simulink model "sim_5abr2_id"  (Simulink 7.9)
settings: Solver=ode45  StartTime=0.0  StopTime=2  RelTol=1e-3  AbsTol=1e-3
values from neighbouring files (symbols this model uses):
  m = 1    [mechanical_system.m]
  s = Lv/norm(Lv)    [pkm1.m]
undefined symbols (not defined in the file or in its folder): deg, kg, mN, N, rad
libraries: mblibv1 x16

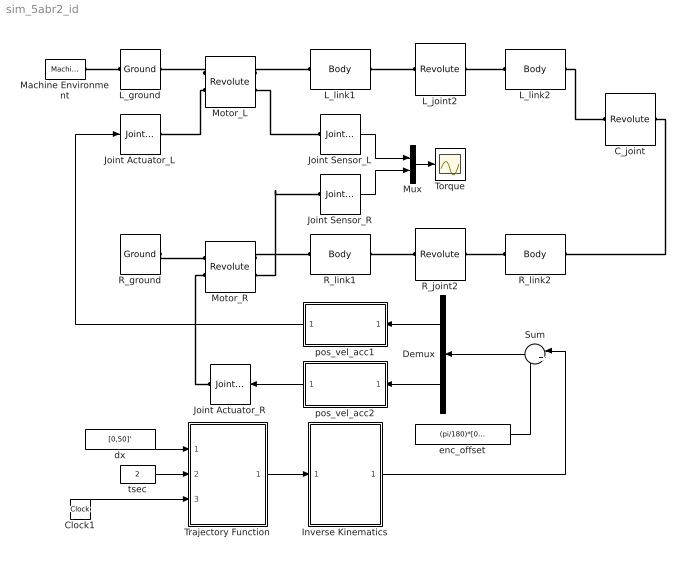
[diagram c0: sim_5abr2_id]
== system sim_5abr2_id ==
  C_joint : mblibv1/Joints/Revolute  LConnTagsString=__newl0  RConnTagsString=__newr0  UpdateFromCAD=off  NumSAPorts=0  CutJoint=off  MarkAsCut=off  Primitives=prismatic  PrimitiveProps=R1$World$[0 0 1]$revolute  DialogClass=JointBlock  R1Axis=[0 0 1]
  Clock1 : Clock
  Demux : Demux  Outputs=2
  Inverse Kinematics : MATLAB Function  TreatAsAtomicUnit=on
  Joint Actuator_L : mblibv1/Sensors &  Actuators/Joint Actuator  UpdateFromCAD=off  PhysicalDomain=Mechanical  PortType=blob  ActuationStyle=Motion  AngleUnits=rad  ArcVelocityUnits=rad/s  ArcAccelerationUnits=rad/s^2  CoordPositionUnits=m  VelocityUnits=m/s  AccelerationUnits=m/s^2  ForceUnits=N  TorqueUnits=N*m  ActiveIO=on  Width=3  DialogClass=MechanicalActuatorBlock  Primitive=R1  ReferenceFrame=Absolute (World)
  Joint Actuator_R : mblibv1/Sensors &  Actuators/Joint Actuator  UpdateFromCAD=off  PhysicalDomain=Mechanical  PortType=blob  ActuationStyle=Motion  AngleUnits=rad  ArcVelocityUnits=rad/s  ArcAccelerationUnits=rad/s^2  CoordPositionUnits=m  VelocityUnits=m/s  AccelerationUnits=m/s^2  ForceUnits=N  TorqueUnits=N*m  ActiveIO=on  Width=3  DialogClass=MechanicalActuatorBlock  Primitive=R1  ReferenceFrame=Absolute (World)
  Joint Sensor_L : mblibv1/Sensors &  Actuators/Joint Sensor  UpdateFromCAD=off  PhysicalDomain=Mechanical  PortType=blob  Muxed=on  Pose=off  Angle=off  AngleUnits=deg  ArcVelocity=off  ArcVelocityUnits=deg/s  ArcAcceleration=off  ArcAccelerationUnits=deg/s^2  CoordPosition=on  CoordPositionUnits=m  Velocity=off  VelocityUnits=m/s  Acceleration=off  AccelerationUnits=m/s^2  Quaternion=on  QuaternionDT=off  QuaternionDDT=off  QuaternionUnits=off  OutputVector=[1]  ActiveIO=on  Width=1  DialogClass=MechanicalSensorBlock  Primitive=R1  Force=off  ForceUnits=N  Torque=on  TorqueUnits=mN*m  ReferenceFrame=Absolute (World)  ReactionSensedSide=Base  ReactionReferenceFrame=Absolute (World)  ReactionForce=off  ReactionForceUnits=N  ReactionMoment=off  ReactionMomentUnits=N*m
  Joint Sensor_R : mblibv1/Sensors &  Actuators/Joint Sensor  UpdateFromCAD=off  PhysicalDomain=Mechanical  PortType=blob  Muxed=on  Pose=off  Angle=off  AngleUnits=deg  ArcVelocity=off  ArcVelocityUnits=deg/s  ArcAcceleration=off  ArcAccelerationUnits=deg/s^2  CoordPosition=on  CoordPositionUnits=m  Velocity=off  VelocityUnits=m/s  Acceleration=off  AccelerationUnits=m/s^2  Quaternion=on  QuaternionDT=off  QuaternionDDT=off  QuaternionUnits=off  OutputVector=[1]  ActiveIO=on  Width=1  DialogClass=MechanicalSensorBlock  Primitive=R1  Force=off  ForceUnits=N  Torque=on  TorqueUnits=mN*m  ReferenceFrame=Absolute (World)  ReactionSensedSide=Base  ReactionReferenceFrame=Absolute (World)  ReactionForce=off  ReactionForceUnits=N  ReactionMoment=off  ReactionMomentUnits=N*m
  L_ground : mblibv1/Bodies/Ground  UpdateFromCAD=off  LeftPortType=env  RightPortType=workingframe  PhysicalDomain=Mechanical  DialogClass=GroundBlock  CoordPosition=[0 0 0]  CoordPositionUnits=cm  StateVectorMgrId=-1  MachineId=[0 0]  ShowEnvPort=on
  L_joint2 : mblibv1/Joints/Revolute  LConnTagsString=__newl0  RConnTagsString=__newr0  UpdateFromCAD=off  NumSAPorts=0  CutJoint=off  MarkAsCut=off  Primitives=prismatic  PrimitiveProps=R1$World$[0 0 1]$revolute  DialogClass=JointBlock  R1Axis=[0 0 1]
  L_link1 : mblibv1/Bodies/Body  LConnTagsString=CS1  RConnTagsString=CS2  UpdateFromCAD=off  DialogClass=MechanicalBodyBlock  Mass=0.053  MassUnits=kg  InertiaUnits=kg*m^2  Inertia=[0.000110621 0 0; 0 0.000110621 0; 0 0 0]  Shape=Cylinder  ShapeDims=[1 1]  ShapeUnits=m  ShapeUse=false  Density=1  DensityUnits=kg/m^3  DensityUse=false  GraphicsMode=MACHINE_DEFAULT  BodyColorSelMode=MACHINE_DEFAULT  BodyColor=[1 0 0]  AttachedToCS=CG  CG=Left$CG$[0.05311 0 0]$CS1$CS1$m$[0 0 0]$Euler X-Y-Z$deg$WORLD$false$none  WorkingFrames=Left$CS1$[0 0 0]$World$World$m$[0 0 0]$Euler X-Y-Z$deg$WORLD$true$none#Right$CS2$[0.1 0 0]$World$World$m$[0 0 0]$Euler X-Y-Z$deg$WORLD$true$none  CGPos=[0.05311 0 0]  CGRot=[0 0 0]  CS0Pos=[]  CS0Rot=[]  CS1Pos=[0 0 0]  CS1Rot=[0 0 0]  CS2Pos=[0.1 0 0]  CS2Rot=[0 0 0]  CS3Pos=[]  CS3Rot=[]  CS4Pos=[]  CS4Rot=[]  CS5Pos=[]  CS5Rot=[]  CS6Pos=[]  CS6Rot=[]  CS7Pos=[]  CS7Rot=[]  CS8Pos=[]  CS8Rot=[]  CS9Pos=[]  CS9Rot=[]  CS10Pos=[]  CS10Rot=[]  CS11Pos=[]  CS11Rot=[]  CS12Pos=[]  CS12Rot=[]  CS13Pos=[]  CS13Rot=[]  CS14Pos=[]  CS14Rot=[]  CS15Pos=[]  CS15Rot=[]  CS16Pos=[]  CS16Rot=[]  CS17Pos=[]  CS17Rot=[]  CS18Pos=[]  CS18Rot=[]  CS19Pos=[]  CS19Rot=[]  CS20Pos=[]  CS20Rot=[]
  L_link2 : mblibv1/Bodies/Body  LConnTagsString=CS1  RConnTagsString=CS2  UpdateFromCAD=off  DialogClass=MechanicalBodyBlock  Mass=0.054  MassUnits=kg  InertiaUnits=kg*m^2  Inertia=[0.000120188 0 0; 0 0.000120188 0; 0 0 0]  Shape=Cylinder  ShapeDims=[1 1]  ShapeUnits=m  ShapeUse=false  Density=1  DensityUnits=kg/m^3  DensityUse=false  GraphicsMode=MACHINE_DEFAULT  BodyColorSelMode=MACHINE_DEFAULT  BodyColor=[1 0 0]  AttachedToCS=CG  CG=Left$CG$[0 0.05992 0]$CS1$CS1$m$[0 0 0]$Euler X-Y-Z$deg$WORLD$false$none  WorkingFrames=Left$CS1$[0.1 0 0]$World$World$m$[0 0 0]$Euler X-Y-Z$deg$WORLD$true$none#Right$CS2$[0.1 0.1 0]$World$World$m$[0 0 0]$Euler X-Y-Z$deg$WORLD$true$none#Left$CS3$[0.1 0.128 0]$World$World$m$[0 0 0]$Euler X-Y-Z$deg$WORLD$false$none  CGPos=[0 0.05992 0]  CGRot=[0 0 0]  CS0Pos=[]  CS0Rot=[]  CS1Pos=[0.1 0 0]  CS1Rot=[0 0 0]  CS2Pos=[0.1 0.1 0]  CS2Rot=[0 0 0]  CS3Pos=[0.1 0.128 0]  CS3Rot=[0 0 0]  CS4Pos=[]  CS4Rot=[]  CS5Pos=[]  CS5Rot=[]  CS6Pos=[]  CS6Rot=[]  CS7Pos=[]  CS7Rot=[]  CS8Pos=[]  CS8Rot=[]  CS9Pos=[]  CS9Rot=[]  CS10Pos=[]  CS10Rot=[]  CS11Pos=[]  CS11Rot=[]  CS12Pos=[]  CS12Rot=[]  CS13Pos=[]  CS13Rot=[]  CS14Pos=[]  CS14Rot=[]  CS15Pos=[]  CS15Rot=[]  CS16Pos=[]  CS16Rot=[]  CS17Pos=[]  CS17Rot=[]  CS18Pos=[]  CS18Rot=[]  CS19Pos=[]  CS19Rot=[]  CS20Pos=[]  CS20Rot=[]
  Machine Environment : mblibv1/Bodies/Machine Environment  PortType=env  PhysicalDomain=Mechanical  DialogTemplateClass=MECH.MachineEnvironment  SyncWhenCopied=off  Gravity=[0 -9.81 0]  GravityUnits=m/s^2  GravityAsSignal=off  Dimensionality=Auto-detect  AnalysisType=Forward dynamics  LinearAssemblyTolerance=1e-3  LinearAssemblyToleranceUnits=m  AngularAssemblyTolerance=1e-3  AngularAssemblyToleranceUnits=rad  ConstraintSolverType=Stabilizing  ConstraintRelTolerance=1e-4  ConstraintAbsTolerance=1e-4  UseRobustSingularityHandling=off  RedundancyAnalysisToleranceType=Automatically select tolerance  RedundancyAnalysisTolerance=1e-14  StatePerturbationType=Fixed  PerturbationSize=1e-5  VisualizeMachine=on  BodyVisualizationType=Use model default body geometries  BodyColorSelMode=Use model default  DefaultBodyColor=[1 0 0]
  Motor_L : mblibv1/Joints/Revolute  LConnTagsString=__newl0|SA1  RConnTagsString=__newr0|SA1  UpdateFromCAD=off  NumSAPorts=2  CutJoint=off  MarkAsCut=off  Primitives=prismatic  PrimitiveProps=R1$World$[0 0 1]$revolute  DialogClass=JointBlock  R1Axis=[0 0 1]
  Motor_R : mblibv1/Joints/Revolute  LConnTagsString=__newl0|SA1  RConnTagsString=__newr0|SA1  UpdateFromCAD=off  NumSAPorts=2  CutJoint=off  MarkAsCut=off  Primitives=prismatic  PrimitiveProps=R1$World$[0 0 1]$revolute  DialogClass=JointBlock  R1Axis=[0 0 1]
  Mux : Mux  Inputs=2
  R_ground : mblibv1/Bodies/Ground  UpdateFromCAD=off  LeftPortType=env  RightPortType=workingframe  PhysicalDomain=Mechanical  DialogClass=GroundBlock  CoordPosition=[0.2 0 0]  CoordPositionUnits=m  StateVectorMgrId=-1  MachineId=[0 0]  ShowEnvPort=off
  R_joint2 : mblibv1/Joints/Revolute  LConnTagsString=__newl0  RConnTagsString=__newr0  UpdateFromCAD=off  NumSAPorts=0  CutJoint=off  MarkAsCut=off  Primitives=prismatic  PrimitiveProps=R1$World$[0 0 1]$revolute  DialogClass=JointBlock  R1Axis=[0 0 1]
  R_link1 : mblibv1/Bodies/Body  LConnTagsString=CS1  RConnTagsString=CS2  UpdateFromCAD=off  DialogClass=MechanicalBodyBlock  Mass=0.061  MassUnits=kg  InertiaUnits=kg*m^2  Inertia=[0.000134303 0 0; 0 0.000134303 0; 0 0 0]  Shape=Cylinder  ShapeDims=[1 1]  ShapeUnits=m  ShapeUse=false  Density=1  DensityUnits=kg/m^3  DensityUse=false  GraphicsMode=MACHINE_DEFAULT  BodyColorSelMode=MACHINE_DEFAULT  BodyColor=[1 0 0]  AttachedToCS=CG  CG=Left$CG$[0 0.04569 0]$CS1$CS1$m$[0 0 0]$Euler X-Y-Z$deg$WORLD$false$none  WorkingFrames=Left$CS1$[0.2 0 0]$World$World$m$[0 0 0]$Euler X-Y-Z$deg$WORLD$true$none#Right$CS2$[0.2 0.1 0]$World$World$m$[0 0 0]$Euler X-Y-Z$deg$WORLD$true$none  CGPos=[0 0.04569 0]  CGRot=[0 0 0]  CS0Pos=[]  CS0Rot=[]  CS1Pos=[0.2 0 0]  CS1Rot=[0 0 0]  CS2Pos=[0.2 0.1 0]  CS2Rot=[0 0 0]  CS3Pos=[]  CS3Rot=[]  CS4Pos=[]  CS4Rot=[]  CS5Pos=[]  CS5Rot=[]  CS6Pos=[]  CS6Rot=[]  CS7Pos=[]  CS7Rot=[]  CS8Pos=[]  CS8Rot=[]  CS9Pos=[]  CS9Rot=[]  CS10Pos=[]  CS10Rot=[]  CS11Pos=[]  CS11Rot=[]  CS12Pos=[]  CS12Rot=[]  CS13Pos=[]  CS13Rot=[]  CS14Pos=[]  CS14Rot=[]  CS15Pos=[]  CS15Rot=[]  CS16Pos=[]  CS16Rot=[]  CS17Pos=[]  CS17Rot=[]  CS18Pos=[]  CS18Rot=[]  CS19Pos=[]  CS19Rot=[]  CS20Pos=[]  CS20Rot=[]
  R_link2 : mblibv1/Bodies/Body  LConnTagsString=CS1  RConnTagsString=CS2  UpdateFromCAD=off  DialogClass=MechanicalBodyBlock  Mass=0.045  MassUnits=kg  InertiaUnits=kg*m^2  Inertia=[0.000090992 0 0; 0 0.000090992 0; 0 0 0]  Shape=Cylinder  ShapeDims=[1 1]  ShapeUnits=m  ShapeUse=false  Density=1  DensityUnits=kg/m^3  DensityUse=false  GraphicsMode=MACHINE_DEFAULT  BodyColorSelMode=MACHINE_DEFAULT  BodyColor=[1 0 0]  AttachedToCS=CG  CG=Left$CG$[-0.05 0 0]$CS1$CS1$m$[0 0 0]$Euler X-Y-Z$deg$WORLD$false$none  WorkingFrames=Left$CS1$[0.2 0.1 0]$World$World$m$[0 0 0]$Euler X-Y-Z$deg$WORLD$true$none#Right$CS2$[0.1 0.1 0]$World$World$m$[0 0 0]$Euler X-Y-Z$deg$WORLD$true$none  CGPos=[-0.05 0 0]  CGRot=[0 0 0]  CS0Pos=[]  CS0Rot=[]  CS1Pos=[0.2 0.1 0]  CS1Rot=[0 0 0]  CS2Pos=[0.1 0.1 0]  CS2Rot=[0 0 0]  CS3Pos=[]  CS3Rot=[]  CS4Pos=[]  CS4Rot=[]  CS5Pos=[]  CS5Rot=[]  CS6Pos=[]  CS6Rot=[]  CS7Pos=[]  CS7Rot=[]  CS8Pos=[]  CS8Rot=[]  CS9Pos=[]  CS9Rot=[]  CS10Pos=[]  CS10Rot=[]  CS11Pos=[]  CS11Rot=[]  CS12Pos=[]  CS12Rot=[]  CS13Pos=[]  CS13Rot=[]  CS14Pos=[]  CS14Rot=[]  CS15Pos=[]  CS15Rot=[]  CS16Pos=[]  CS16Rot=[]  CS17Pos=[]  CS17Rot=[]  CS18Pos=[]  CS18Rot=[]  CS19Pos=[]  CS19Rot=[]  CS20Pos=[]  CS20Rot=[]
  Sum : Sum  Inputs=|+-
  Torque : Scope
  Trajectory Function : MATLAB Function  TreatAsAtomicUnit=on
  dx : Constant  Value=[0,50]'  SampleTime=-1
  enc_offset : Constant  Value=(pi/180)*[0,90]'
  pos_vel_acc1 : Subsystem
  pos_vel_acc2 : Subsystem
  tsec : Constant  Value=2  SampleTime=-1
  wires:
  pos_vel_acc2/1(Motion2) -> Joint Actuator_R/1
  pos_vel_acc1/1(Motion1) -> Joint Actuator_L/1
  Inverse Kinematics/1(thd) -> Sum/1
  Trajectory Function/1(xd) -> Inverse Kinematics/1(xd)
  Clock1/1 -> Trajectory Function/3(tout)
  tsec/1 -> Trajectory Function/2(tsec)
  dx/1 -> Trajectory Function/1(dx)
  Demux/1 -> pos_vel_acc1/1(In1)
  Demux/2 -> pos_vel_acc2/1(In1)
  enc_offset/1 -> Sum/2
  Sum/1 -> Demux/1
  Mux/1 -> Torque/1
  Joint Sensor_L/1 -> Mux/1
  Joint Sensor_R/1 -> Mux/2
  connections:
  L_joint2/RConn1 -- L_link2/LConn1
  Motor_L/LConn1 -- L_ground/RConn1
  L_joint2/LConn1 -- L_link1/RConn1
  Motor_L/RConn1 -- L_link1/LConn1
  R_joint2/RConn1 -- R_link2/LConn1
  R_joint2/LConn1 -- R_link1/RConn1
  L_link2/RConn1 -- C_joint/LConn1
  C_joint/RConn1 -- R_link2/RConn1
  Motor_R/RConn1 -- R_link1/LConn1
  R_ground/RConn1 -- Motor_R/LConn1
  Motor_L/RConn2 -- Joint Sensor_L/LConn1
  Motor_R/RConn2 -- Joint Sensor_R/LConn1
  Motor_L/LConn2 -- Joint Actuator_L/RConn1
  Motor_R/LConn2 -- Joint Actuator_R/RConn1
  Machine Environment/RConn1 -- L_ground/LConn1

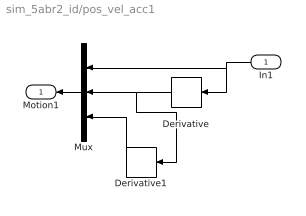
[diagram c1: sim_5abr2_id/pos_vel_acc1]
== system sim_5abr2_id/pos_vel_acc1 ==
  In1 : Inport
  Derivative : Derivative
  Derivative1 : Derivative
  Mux : Mux  Inputs=3
  Motion1 : Outport
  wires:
  Mux/1 -> Motion1/1
  Derivative/1 -> Mux/2, Derivative1/1
  Derivative1/1 -> Mux/3
  In1/1 -> Mux/1, Derivative/1

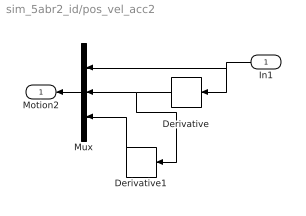
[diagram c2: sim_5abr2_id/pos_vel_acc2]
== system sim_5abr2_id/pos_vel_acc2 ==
  In1 : Inport
  Derivative : Derivative
  Derivative1 : Derivative
  Mux : Mux  Inputs=3
  Motion2 : Outport
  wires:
  Mux/1 -> Motion2/1
  Derivative/1 -> Mux/2, Derivative1/1
  Derivative1/1 -> Mux/3
  In1/1 -> Mux/1, Derivative/1

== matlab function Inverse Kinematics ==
function thd  = fcn(xd)

persistent index thd_p
persistent th3_p th4_p

% Initializing Variables %
if isempty(index), index=0; end
if isempty(thd_p), thd_p=(pi/180)*[0,90]'; end
if isempty(th3_p), th3_p=0; end
if isempty(th4_p), th4_p=0; end

% Kinematic Parameters %
L1=200; L2=100; L3=100; L4=100; L5=100; L6=28;

w_index=1;  % In workspace %

% (1) Left Side 2-DOF Arm %
px=xd(1,1); py=xd(2,1);
k1=(px^2+py^2-L2^2-(L3+L6)^2)/(2*L2*(L3+L6));
if abs(k1)<=1
    th3=+acos(k1);  % Note the sign %
else
    w_index=-1;
    th3=th3_p;
end

DEL1=L2^2+(L3+L6)^2+2*L2*(L3+L6)*cos(th3);
cth2=(px*(L2+(L3+L6)*cos(th3))+py*(L3+L6)*sin(th3))/DEL1;
sth2=(-px*(L3+L6)*sin(th3)+py*(L2+(L3+L6)*cos(th3)))/DEL1;
th2=atan2(sth2,cth2);

% (2) Right Side 2-DOF Arm %
cx=px-L6*cos(th2+th3)-L1; cy=py-L6*sin(th2+th3);
k2=(cx^2+cy^2-L5^2-L4^2)/(2*L5*L4);
if abs(k2)<=1
    th4=acos(k2);
else
    w_index=-2;
    th4=th4_p;
end

DEL2=L5^2+L4^2+2*L5*L4*cos(th4);
cth5=(cx*(L5+L4*cos(th4))+cy*L4*sin(th4))/DEL2;
sth5=(-cx*L4*sin(th4)+cy*(L5+L4*cos(th4)))/DEL2;
th5=atan2(sth5,cth5);

% Result %
if w_index==1
    thd=[th2, th5]';
else
    thd=thd_p;
end

% Save the current value %
thd_p=thd;
th3_p=th3; th4_p=th4;

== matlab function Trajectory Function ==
function xd = fcn(dx, tsec, tout)

MAX_CH=2;       % Two Actuators %

% Initializing Variables %
xd=zeros(MAX_CH,1);
x0=[100, 128]';

[c] = coeff_3rd(x0, zeros(MAX_CH,1), x0+dx, zeros(MAX_CH,1), tsec);
for ch=1:MAX_CH
    xd(ch,1)=c(ch,1)+c(ch,2)*tout+c(ch,3)*tout^2+c(ch,4)*tout^3;    
end

function [c] = coeff_3rd(sp, sv, ep, ev, tsec)
MAX_CH=2;
c=zeros(MAX_CH,4);
for ch=1:MAX_CH
    c(ch,1)=sp(ch,1);
    c(ch,2)=sv(ch,1);
    c(ch,3)=(3.0*(ep(ch,1)-sp(ch,1))-(2.0*sv(ch,1)+ev(ch,1))*tsec)/(tsec*tsec);
    c(ch,4)=(-2.0*(ep(ch,1)-sp(ch,1))+(sv(ch,1)+ev(ch,1))*tsec)/(tsec*tsec*tsec);
end
